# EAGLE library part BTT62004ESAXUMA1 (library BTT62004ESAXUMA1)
Quad Channel Smart High-Side Power Switch Source: Datasheet
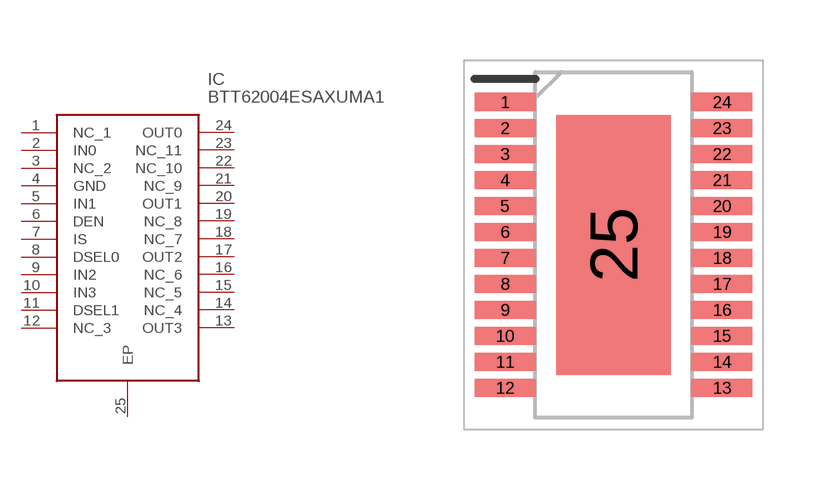
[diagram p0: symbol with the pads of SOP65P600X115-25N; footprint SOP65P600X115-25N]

Designator prefix IC

## BTT62004ESAXUMA1 (Description: Quad Channel Smart High-Side Power Switch; Height: 1.15mm; Manufacturer_Name: Infineon; Manufacturer_Part_Number: BTT62004ESAXUMA1; Mouser_Part_Number: 726-BTT62004ESAXUMA1; Mouser_Price-Stock: https://www.mouser.co.uk/ProductDetail/Infineon-Technologies/BTT62004ESAXUMA1?qs=unwgFEO1A6tpV1sLwJtTRA%3D%3D)  [SOP65P600X115-25N]
1  NC_1
2  IN0
3  NC_2
4  GND
5  IN1
6  DEN
7  IS
8  DSEL0
9  IN2
10  IN3
11  DSEL1
12  NC_3
13  OUT3
14  NC_4
15  NC_5
16  NC_6
17  OUT2
18  NC_7
19  NC_8
20  OUT1
21  NC_9
22  NC_10
23  NC_11
24  OUT0
25  EP

## Footprint SOP65P600X115-25N (pad centres in mm)
PG-TSDSO-24-1
smd 1.525 x 0.45: 1 -2.712,3.575; 2 -2.712,2.925; 3 -2.712,2.275; 4 -2.712,1.625; 5 -2.712,0.975; 6 -2.712,0.325; 7 -2.712,-0.325; 8 -2.712,-0.975; 9 -2.712,-1.625; 10 -2.712,-2.275; 11 -2.712,-2.925; 12 -2.712,-3.575; 13 2.712,-3.575; 14 2.712,-2.925; 15 2.712,-2.275; 16 2.712,-1.625; 17 2.712,-0.975; 18 2.712,-0.325; 19 2.712,0.325; 20 2.712,0.975; 21 2.712,1.625; 22 2.712,2.275; 23 2.712,2.925; 24 2.712,3.575
smd 2.87 x 6.5: 25 0,0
